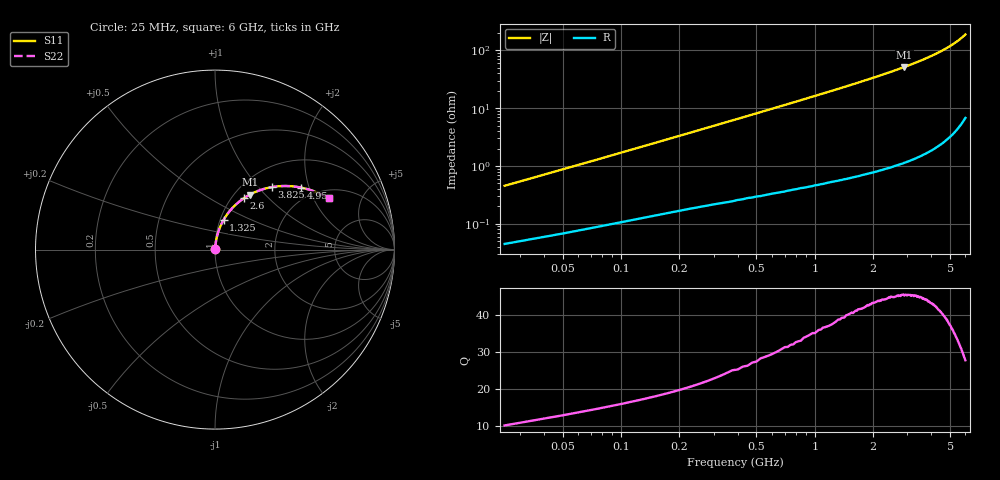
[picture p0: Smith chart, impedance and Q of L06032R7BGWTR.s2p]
!	AVX Thin Film Operation
!	Date:	March	2003
!	Description: Accu-L® Series Thin Film SMD RF Inductors
!	Part Number: L06032R7BGWTR
!	25MHz-6GHz
!	Serial	Measurements
#	mhz	S	db	R	50
!	S11	S11	S21	S21	S12	S12	S22	S22
!	dB	Phase	dB	Phase	dB	Phase	dB	Phase
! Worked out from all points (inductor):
!   240 points, 25 MHz to 6 GHz, reference 50 ohm
!   read as 1/Y11, port 2 shorted: L = 2.74 nH near 50 MHz
!   highest Q = 45.6 at 2.9 GHz (marker M1), where L = 2.84 nH
!   S11 on the Smith chart (normalised r, x): 25 MHz: 1.00, +0.01; 1.325 GHz: 1.04, +0.35; 2.6 GHz: 1.13, +0.73; 3.825 GHz: 1.32, +1.18; 4.95 GHz: 1.67, +1.77; 6 GHz: 2.39, +2.64
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25  -48.34 83.0  -0.00 -0.3  -0.00 -0.3  -48.34 83.0
50  -42.70 84.0  -0.01 -0.6  -0.01 -0.6  -42.70 84.0
75  -39.37 84.3  -0.01 -0.9  -0.01 -0.9  -39.37 84.3
100  -37.00 84.5  -0.01 -1.1  -0.01 -1.1  -37.00 84.5
125  -35.15 84.5  -0.01 -1.4  -0.01 -1.4  -35.15 84.5
175  -32.34 84.4  -0.02 -2.0  -0.02 -2.0  -32.34 84.4
225  -30.24 84.1  -0.02 -2.5  -0.02 -2.5  -30.24 84.1
275  -28.56 83.8  -0.02 -3.1  -0.02 -3.1  -28.56 83.8
400  -25.41 82.9  -0.04 -4.4  -0.04 -4.4  -25.41 82.9
575  -22.35 81.3  -0.05 -6.3  -0.05 -6.3  -22.35 81.3
775  -19.82 79.4  -0.08 -8.4  -0.08 -8.4  -19.82 79.4
1025  -17.46 76.9  -0.12 -11.1  -0.12 -11.1  -17.46 76.9
1325  -15.30 73.9  -0.18 -14.3  -0.18 -14.3  -15.30 73.9
2025  -11.74 66.7  -0.36 -21.7  -0.36 -21.7  -11.74 66.7
2600  -9.68 60.7  -0.57 -27.8  -0.57 -27.8  -9.68 60.7
2900  -8.79 57.5  -0.70 -31.0  -0.70 -31.0  -8.79 57.5
3025  -8.44 56.2  -0.75 -32.3  -0.75 -32.3  -8.44 56.2
3825  -6.57 47.8  -1.19 -40.8  -1.19 -40.8  -6.57 47.8
4025  -6.17 45.7  -1.31 -42.9  -1.31 -42.9  -6.17 45.7
4950  -4.58 35.8  -2.01 -52.7  -2.01 -52.7  -4.58 35.8
5025  -4.46 35.0  -2.07 -53.5  -2.07 -53.5  -4.46 35.0
6000  -3.16 24.3  -3.07 -64.1  -3.07 -64.1  -3.16 24.3
